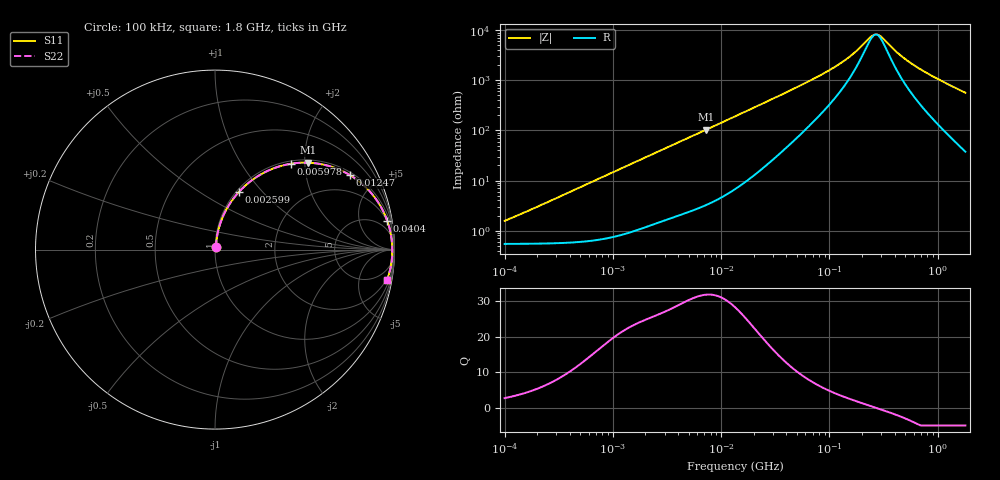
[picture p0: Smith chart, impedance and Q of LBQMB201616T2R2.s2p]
! LBQMB201616T2R2  S-PARAMETER MODEL  ( General Type )
! Model Generated by TAIYO YUDEN Corporation (http://www.ty-top.com)
! Version 1.0
! TAIYO YUDEN Control No. 191025NI43SB-FBB
! Copyright(c) 2019 TAIYO YUDEN CO.,LTD. All Rights Reserved.
! Product Description (link to TY-COMPAS)
! https://ds.yuden.co.jp/TYCOMPAS/or/detail?pn=LBQMB201616T2R2J&u=M
! Products Name : Inductors
! Characteristics :
!  Inductance : 2.2 uH , SRF(min) : 75 MHz , DC Resistance(max) : 0.702 Ohm , Rated Current : 340 mA
!  Case Size : 2.0 x 1.6 / 0.079 x 0.063 [mm/inch] , Thickness : 1.6 / 0.063 [mm/inch]
!  (Conditions: Temperature = 25 degC , DC Bias Current/Voltage = 0A / 0V)
! External Node Assignments :
!  1  o---GGG---o  2
! GND o---------o GND
! Frequency Range : 0.1MHz  -  1800MHz  [ 402 STEP ]
# MHz S RI R 50
! Freq[MHz].  S11 Real  S11 Imag  S21 Real  S21 Imag  S12 Real  S12 Imag  S22 Real  S22 Imag
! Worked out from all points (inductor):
!   401 points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, 100 kHz to 1.8 GHz, reference 50 ohm
!   read as one part in series: L = 2.34 uH near 113 kHz
!   highest Q = 31.9 at 7.272 MHz (marker M1), where L = 2.26 uH
!   self-resonance near 268.6 MHz
!   S11 on the Smith chart (normalised r, x): 100 kHz: 1.01, +0.03; 2.599 MHz: 1.03, +0.75; 5.978 MHz: 1.05, +1.70; 12.47 MHz: 1.12, +3.54; 40.4 MHz: 2, +12; 1.8 GHz: 2, -11
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0.1  0.00561 0.0145  0.9944 -0.0145  0.9944 -0.0145  0.00561 0.0145
0.516129  0.0116 0.0744  0.9884 -0.0744  0.9884 -0.0744  0.0116 0.0744
1.341675  0.0447 0.1853  0.9553 -0.1853  0.9553 -0.1853  0.0447 0.1853
2.59943  0.1328 0.3208  0.8672 -0.3208  0.8672 -0.3208  0.1328 0.3208
2.66389  0.138 0.3265  0.862 -0.3265  0.862 -0.3265  0.138 0.3265
3.942096  0.2495 0.4157  0.7505 -0.4157  0.7505 -0.4157  0.2495 0.4157
5.97828  0.423 0.4783  0.577 -0.4783  0.577 -0.4783  0.423 0.4783
7.272466  0.5165 0.4843  0.4835 -0.4843  0.4835 -0.4843  0.5165 0.4843
12.46584  0.7507 0.4158  0.2493 -0.4158  0.2493 -0.4158  0.7507 0.4158
13.41641  0.776 0.3997  0.224 -0.3997  0.224 -0.3997  0.776 0.3997
21.89777  0.8958 0.2828  0.1042 -0.2828  0.1042 -0.2828  0.8958 0.2828
40.39749  0.9592 0.1619  0.0408 -0.1619  0.0408 -0.1619  0.9592 0.1619
69.24595  0.9784 0.0923  0.0216 -0.0923  0.0216 -0.0923  0.9784 0.0923
140.897  0.9862 0.0357  0.0138 -0.0357  0.0138 -0.0357  0.9862 0.0357
253.6402  0.988 0.00299  0.012 -0.00299  0.012 -0.00299  0.988 0.00299
272.9811  0.988 -0.000847  0.012 0.000847  0.012 0.000847  0.988 -0.000847
293.7968  0.9881 -0.0047  0.0119 0.0047  0.0119 0.0047  0.9881 -0.0047
357.3983  0.988 -0.0152  0.012 0.0152  0.012 0.0152  0.988 -0.0152
467.921  0.9873 -0.0307  0.0127 0.0307  0.0127 0.0307  0.9873 -0.0307
659.3364  0.9855 -0.0537  0.0145 0.0537  0.0145 0.0537  0.9855 -0.0537
1050.104  0.9791 -0.0954  0.0209 0.0954  0.0209 0.0954  0.9791 -0.0954
1800  0.959 -0.1676  0.041 0.1676  0.041 0.1676  0.959 -0.1676
